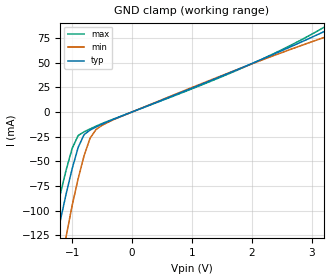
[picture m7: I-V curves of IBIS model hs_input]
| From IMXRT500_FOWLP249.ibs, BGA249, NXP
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[Model] hs_input
|   Model hs_input
| Library cells for typ/min/max conditions are connected as defined below:
|  pad_usbdp - External Pad
|  d_dmpulldn - gnda
|  d_dppulldn - gnda
|  d_sw1_neg - gnda
|  d_sw1_pos - gnda
|  d_sw2_neg - gnda
|  d_sw2_pos - gnda
|  gnda - gnda
|  pad_usb_vss - pad_usb_vss
|  usb2_reg_tx_fs_hiz - gnda
|  usb2_reg_tx_hs_term - gnda
|  usb2_reg_tx_hs_xcvr - vddd
|  usb2_reg_tx_ls_en - gnda
|  usbphy_d2a_txhsactive - gnda
|  vddb - vddb
|  vddd - vddd
| All other pins connected to ground
Model_type Input
Vinl =   0.2100V
Vinh =   0.1900V
C_comp   2.8431pF   2.6338pF   3.0727pF
[Temperature Range]   27.0000   0.1250k   -40.0000
[Voltage Range]   3.1500V   3.0000V   3.3000V
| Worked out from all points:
|   GND clamp passes 1 mA (typ) near -0.04 V on its own axis
[GND_clamp]
|Voltage   I(typ)   I(min)   I(max)
-3.3V     -1.789A    -1.871A    -1.71A
-1.4V     -174.1mA   -255.4mA   -141.3mA
-1.3V     -140.9mA   -205.5mA   -111.5mA
-1.2V     -110.9mA   -162.8mA   -83.93mA
-1.1V     -83.02mA   -126.2mA   -58.78mA
-1V       -57.6mA    -94.84mA   -37mA
-900mV    -35.99mA   -67.67mA   -23.9mA
-800mV    -22.89mA   -44.23mA   -20.13mA
-700mV    -18.35mA   -26.5mA    -17.17mA
-600mV    -15.22mA   -17.69mA   -14.34mA
1.8V      44.02mA    44.06mA    43.55mA
3.2V      81.33mA    75.42mA    85.67mA
